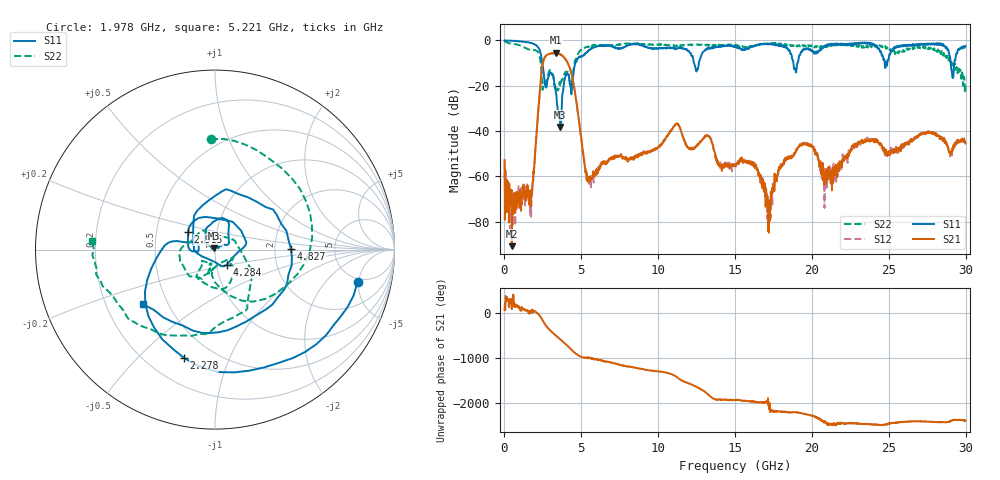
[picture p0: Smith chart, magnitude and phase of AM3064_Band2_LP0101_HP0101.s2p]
# Hz S DB R 50.0
!freq dBS11 angS11 dBS21 angS21 dBS12 angS12 dBS22 angS22
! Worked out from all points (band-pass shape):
!   1600 points, 10 MHz to 29.98 GHz, reference 50 ohm
!   highest |S21| = -5.47 dB at 3.328 GHz (marker M1); lowest = -90.7 dB at 478.6 MHz (marker M2)
!   |S21| within 3 dB of the highest: 2.561 GHz to 3.99 GHz (1.429 GHz wide, 43.6 % of centre)
!   lowest |S11| = -38.2 dB at 3.628 GHz (marker M3), VSWR 1.03, Z = 49.2 + j0.904 ohm
!   |S11| at or under -10 dB: 2.456 GHz to 4.595 GHz (2.14 GHz wide, 60.7 % of centre); 12.32 GHz to 12.64 GHz (318.8 MHz wide, 2.55 % of centre); 18.8 GHz to 19.05 GHz (251.4 MHz wide, 1.33 % of centre)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
!   |S22| runs from -23.2 to -0.2 dB; largest |S21 - S12| = 0.011
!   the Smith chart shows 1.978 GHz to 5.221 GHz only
!   S11 on the Smith chart (normalised r, x): 1.978 GHz: 4.54, -4.81; 2.278 GHz: 0.35, -0.69; 2.915 GHz: 0.73, +0.15; 4.284 GHz: 1.12, -0.19; 4.827 GHz: 2.46, +0.04; 5.221 GHz: 0.36, -0.30
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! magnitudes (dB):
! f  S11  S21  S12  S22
! 10 MHz  0.0  -52.8  -53.9  -0.2
! 478.6 MHz  -0.1  -90.7  -72.6  -1.4
! 1.697 GHz  -1.1  -69.2  -66.2  -4.2
! 1.978 GHz  -1.8  -51.1  -52.3  -4.2
! 2.278 GHz  -4.1  -24.0  -24.1  -6.9
! 2.915 GHz  -14.9  -6.0  -5.9  -13.4
! 3.328 GHz  -21.9  -5.5  -5.4  -20.9
! 3.628 GHz  -38.2  -6.2  -6.1  -19.8
! 4.284 GHz  -19.4  -13.0  -12.8  -18.1
! 4.827 GHz  -7.5  -34.3  -34.4  -5.4
! 5.015 GHz  -7.2  -44.4  -44.2  -4.1
! 5.221 GHz  -6.0  -55.3  -54.9  -3.3
! 10 GHz  -3.5  -47.1  -47.1  -1.9
! 11.22 GHz  -3.7  -36.6  -36.5  -2.2
! 15 GHz  -2.7  -55.4  -55.0  -1.9
! 16.3 GHz  -2.2  -54.8  -55.2  -2.1
! 17.24 GHz  -1.4  -79.9  -71.2  -1.3
! 18.06 GHz  -2.1  -55.0  -54.2  -1.9
! 19.99 GHz  -4.3  -46.9  -46.9  -2.2
! 20.93 GHz  -2.2  -59.8  -58.8  -2.3
! 25 GHz  -8.1  -50.0  -50.8  -3.3
! 29.98 GHz  -2.4  -45.4  -45.4  -20.3
